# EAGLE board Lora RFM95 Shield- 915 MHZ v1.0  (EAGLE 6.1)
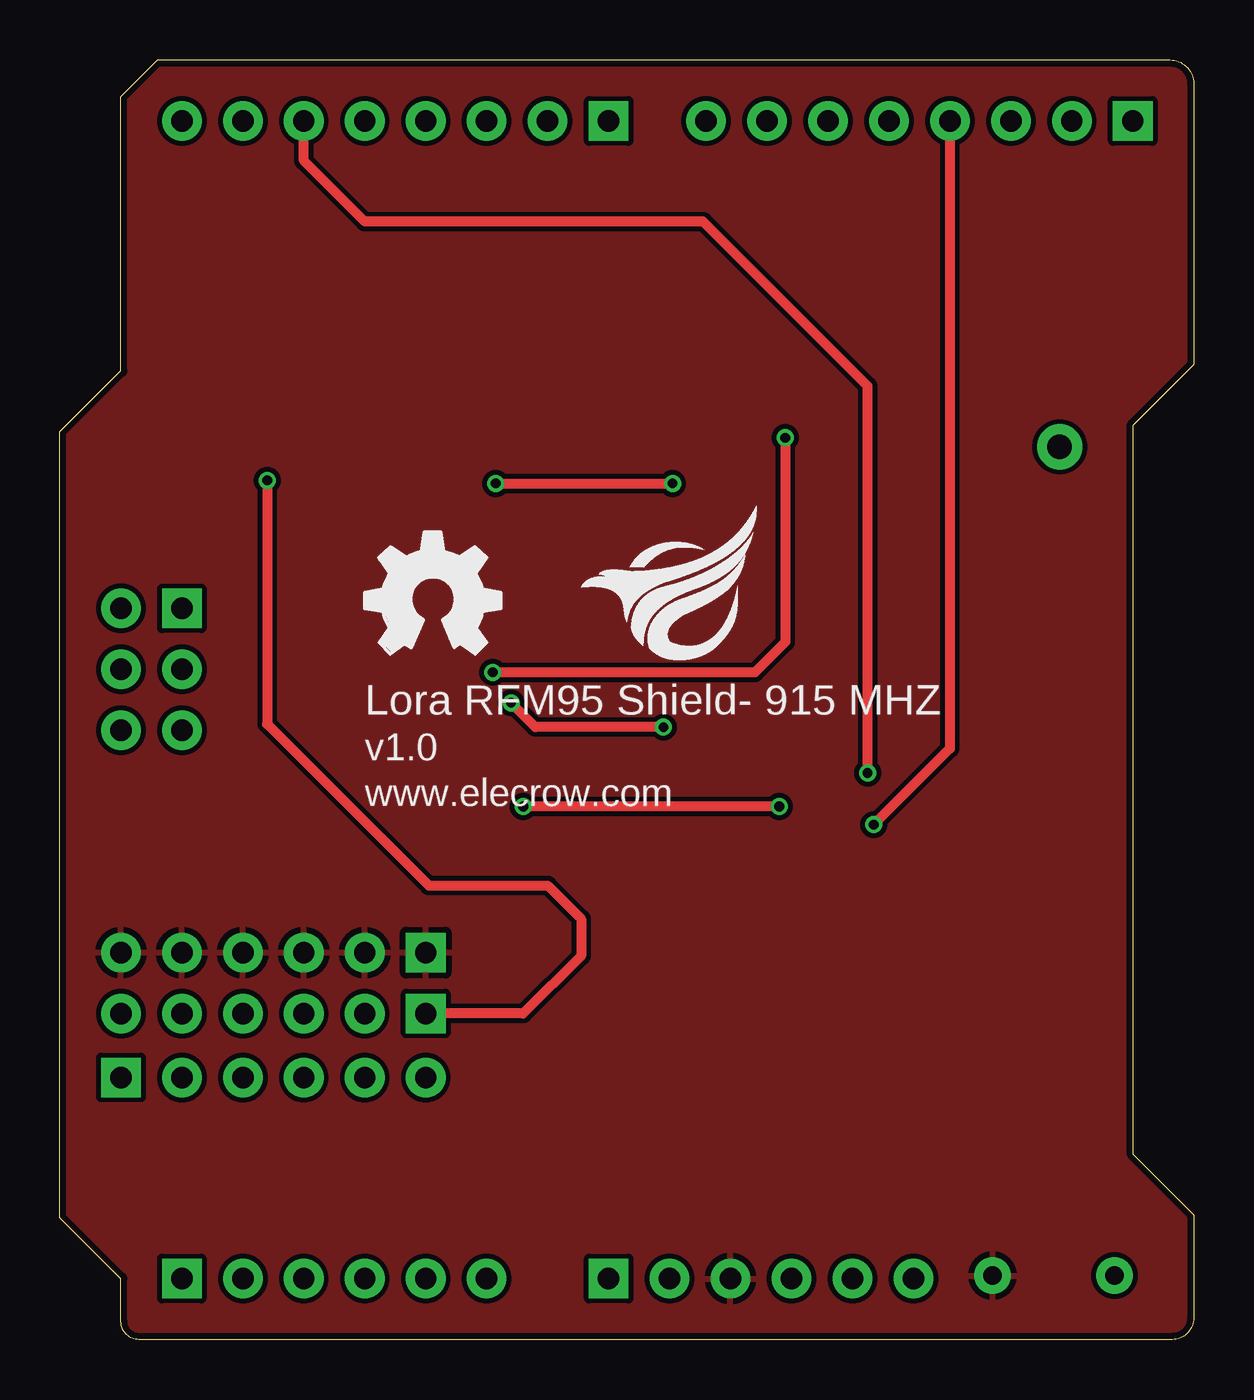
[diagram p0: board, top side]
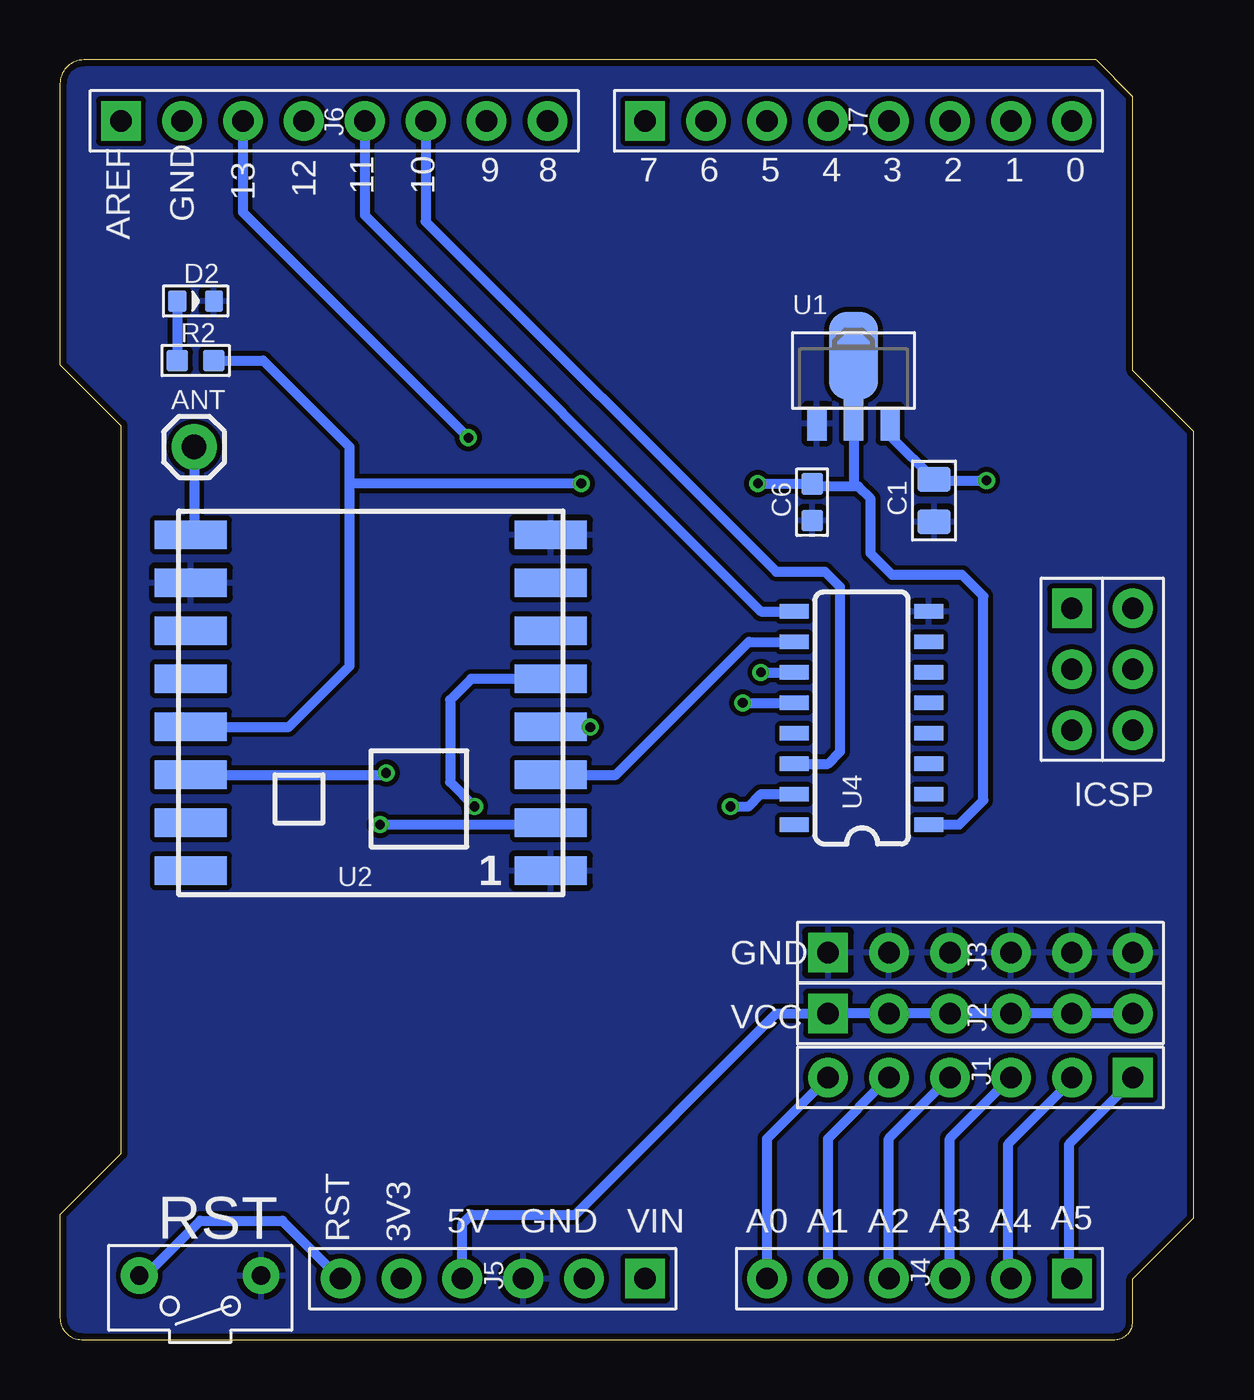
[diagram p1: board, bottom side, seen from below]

Size 47.24 x 53.34 mm. Coordinates in mm from the lower left corner, seen from the top.
Outline: 4.06,53.34 46.25,53.34 arc-90 47.24,52.35 47.24,40.64 44.7,38.1 44.7,7.75 47.24,5.21 47.24,0.9 arc-90 46.35,0 3.28,0 arc-90 2.54,0.74 2.54,2.54 0,5.08 0,37.85 2.54,40.39 2.54,51.82 4.06,53.34
Copper layers (1*16): Top 0.035mm / dielectric 1.5mm / Bottom 0.035mm
Design rules: minimum track width 6mil, minimum drill 12mil, track to track 6mil, track to pad 6mil, pad to pad 6mil, via to via 6mil, smd to smd 0mil, copper to edge 10mil, drill to drill 10mil, minimum pad ring 10mil, minimum via ring 6mil, stop-mask expansion 2mil, vias tented up to drill 100mil, thermal gap 10mil

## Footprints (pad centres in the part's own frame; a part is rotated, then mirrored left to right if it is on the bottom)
1X01 = drill 1.016 pad 1.88: 1 0,0
C0805 = smd 1.016 x 1.397: 1 -0.889,0; 2 0.889,0
C0603 = smd 0.889 x 0.889: 1 -0.762,0; 2 0.762,0
LED-0603 = smd 0.762 x 0.889: + -0.762,0; - 0.762,0
6P-2.54-65/35MIL = drill 0.889 pad 1.651 square: 1 0,6.35 | drill 0.889 pad 1.651: 2 0,3.81; 3 0,1.27; 4 0,-1.27; 5 0,-3.81; 6 0,-6.35
8P-2.54-65/35MIL = drill 0.889 pad 1.651 square: 1 0,8.89 | drill 0.889 pad 1.651: 2 0,6.35; 3 0,3.81; 4 0,1.27; 5 0,-1.27; 6 0,-3.81; 7 0,-6.35; 8 0,-8.89
2X3P-2.54-65/35MIL = drill 0.889 pad 1.651 square: 1 -1.27,2.54 | drill 0.889 pad 1.651: 2 -1.27,0; 3 -1.27,-2.54; 4 1.27,-2.54; 5 1.27,0; 6 1.27,2.54
R0603 = smd 0.889 x 0.889: 1 -0.762,0; 2 0.762,0
2P-7.62X3.56-90D = drill 0.762 pad 1.524: P$1 0,2.54; P$2 0,-2.54
SOT89 = smd 0.8 x 1.4: 1 -1.524,-1.905; 3 1.524,-1.905 | smd 0.8 x 1.9: 2 0,-1.651 | smd 2.032 x 3.65: 4 0,0.94
RFM69HCW-XXXS2 = smd 3 x 1.2: 1 -7.5,7; 2 -7.5,5; 3 -7.5,3; 4 -7.5,1; 5 -7.5,-1; 6 -7.5,-3; 7 -7.5,-5; 8 -7.5,-7; 9 7.5,-7; 10 7.5,-5; 11 7.5,-3; 12 7.5,-1; 13 7.5,1; 14 7.5,3; 15 7.5,5; 16 7.5,7
SO016 = smd 0.6 x 1.2: 1 -4.445,-2.8; 2 -3.175,-2.8; 3 -1.905,-2.8; 4 -0.635,-2.8; 5 0.635,-2.8; 6 1.905,-2.8; 7 3.175,-2.8; 8 4.445,-2.8; 9 4.445,2.8; 10 3.175,2.8; 11 1.905,2.8; 12 0.635,2.8; 13 -0.635,2.8; 14 -1.905,2.8; 15 -3.175,2.8; 16 -4.445,2.8

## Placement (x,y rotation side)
ANT  Antenna  [1X01]  41.66,37.21 0 bottom
C1  10uF  [C0805]  10.82,34.97 90 bottom
C6  0.1uF  [C0603]  15.9,34.91 90 bottom
D2  RED  [LED-0603]  41.59,43.29 0 bottom
J1  [6P-2.54-65/35MIL]  8.89,10.92 270 bottom
J2  [6P-2.54-65/35MIL]  8.89,13.59 90 bottom
J3  [6P-2.54-65/35MIL]  8.89,16.13 90 bottom
J4  [6P-2.54-65/35MIL]  11.43,2.54 270 bottom
J5  [6P-2.54-65/35MIL]  29.21,2.54 270 bottom
J6  [8P-2.54-65/35MIL]  35.81,50.8 90 bottom
J7  [8P-2.54-65/35MIL]  13.97,50.8 90 bottom
J8  [2X3P-2.54-65/35MIL]  3.81,27.94 0 bottom
R2  330  [R0603]  41.59,40.81 0 bottom
RST  K1  [2P-7.62X3.56-90D]  41.4,2.67 270 bottom
U1  [SOT89]  14.18,40.08 0 bottom
U2  RFM69HCW  [RFM69HCW-XXXS2]  34.29,26.54 180 bottom
U4  74HC4050 LVL CONVERTER  [SO016]  13.84,25.91 90 bottom
U$1  [OSHW_FILLX200_NOTEXT]  12.7,28.57 0 top
U$4  [ELECROW_NRW_6]  21.72,28.32 0 top

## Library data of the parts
ANT U4 = SparkFun
C1 C6 D2 R2 RST = Discrete
J1-J8 = Connector
U1 = IC
U2 = mike-temp
U$1 = logo
U$4 = ELECROW

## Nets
3.3V: C6.2 R2.2 U1.2 U1.4 U2.13 U4.1
3V-MOSI: U2.3 U4.10
3V-NSS: U2.5 U4.15
3V-SCK: U2.4 U4.12
5V-MISO: J6.4 U2.2
5V-MOSI: J6.5 U4.9
5V-NSS: J6.6 U4.14
5V-SCK: J6.3 U4.11
DPIO0: J7.6 U2.14
GND: C1.1 C6.1 D2.- J3.1 J3.2 J3.3 J3.4 J3.5 J3.6 J5.3 RST.P$1 U1.1 U2.1 U2.8 U2.10 U4.8
N$1: ANT.1 U2.9
N$2: D2.+ R2.1
N$7: J5.6 RST.P$2
N$10: J5.1
PC0: J1.6 J4.6
PC1: J1.5 J4.5
PC2: J1.4 J4.4
PC3: J1.3 J4.3
PC4: J1.2 J4.2
PC5: J1.1 J4.1
VCC: C1.2 J2.1 J2.2 J2.3 J2.4 J2.5 J2.6 J5.4 U1.3

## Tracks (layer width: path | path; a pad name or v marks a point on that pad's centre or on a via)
3.3V  (via drill 0.41)
  Top 0.406: v18.16,35.69 v25.53,35.69
  Bottom 0.406: U1.4 U1.2 14.18,35.64 14.1,35.56 | 14.1,35.56 13.97,35.56 13.46,35.05 13.46,32.77 12.57,31.88 9.65,31.88 8.76,30.99 8.76,22.48 9.78,21.46 U4.1 | 14.1,35.56 15.79,35.56 C6.2 18.14,35.67 v18.16,35.69 | U2.13 37.7,25.54 35.18,28.07 35.18,35.56 | 35.18,35.56 35.18,37.21 38.78,40.81 R2.2 40.85,40.81 40.89,40.77 | v25.53,35.69 35.05,35.69 35.18,35.56
3V-MOSI
  Bottom 0.406: U2.3 24.08,23.54 18.54,29.08 U4.10
3V-NSS  (via drill 0.41)
  Top 0.406: v29.97,22.23 v19.3,22.23
  Bottom 0.406: U2.5 30.11,27.54 30.99,26.67 30.99,23.24 v29.97,22.23 | v19.3,22.23 18.54,22.23 18.03,22.73 U4.15
3V-SCK  (via drill 0.41)
  Top 0.406: v25.15,25.53 19.81,25.53 v18.8,26.54
  Bottom 0.406: U2.4 25.16,25.54 v25.15,25.53 | v18.8,26.54 U4.12
5V-MISO  (via drill 0.41)
  Top 0.406: J6.4 37.08,24.64 v33.91,21.46
  Bottom 0.406: v33.91,21.46 26.87,21.46 U2.2
5V-MOSI
  Bottom 0.406: J6.5 34.54,46.86 18.03,30.35 U4.9
5V-NSS
  Bottom 0.406: U4.14 15.24,24 14.73,24.51 14.73,31.37 15.37,32 17.4,32 32,46.61 J6.6
5V-SCK  (via drill 0.41)
  Top 0.406: v30.23,37.59 30.23,29.08 28.96,27.81 v18.03,27.81
  Bottom 0.406: 16.51,27.81 U4.11 v18.03,27.81 | J6.3 39.62,46.99 v30.23,37.59
DPIO0  (via drill 0.41)
  Top 0.406: v33.66,23.62 33.66,39.75 26.8,46.61 12.7,46.61 10.16,49.15 J7.6
  Bottom 0.406: U2.14 33.73,23.54 v33.66,23.62
GND
  pour Top (isolate 0.203, rank 6): 47.5,53.34 -0.25,53.34 -0.25,0 47.5,0
  pour Bottom (isolate 0.203, rank 6): 0.51,53.34 -0.13,52.7 -0.13,2.29 2.16,0 47.5,0 47.5,52.7 46.86,53.34
N$1
  Bottom 0.406: ANT.1 41.66,33.4 41.79,33.4 U2.9
N$2
  Bottom 0.406: D2.+ R2.1
N$7
  Bottom 0.406: RST.P$2 43.69,2.67 41.4,4.95 37.97,4.95 J5.6
PC0
  Bottom 0.406: J4.6 17.78,8.38 J1.6
PC1
  Bottom 0.406: J4.5 15.24,8.38 J1.5
PC2
  Bottom 0.406: J4.4 12.7,8.38 J1.4
PC3
  Bottom 0.406: J4.3 10.16,8.38 J1.3
PC4
  Bottom 0.406: J1.2 5.08,10.79 7.75,8.13 7.75,2.67 J4.2
PC5
  Bottom 0.406: J1.1 2.54,10.79 5.21,8.13 5.21,2.67 J4.1
VCC  (via drill 0.41)
  Top 0.406: v8.64,35.81 8.64,25.65 15.37,18.92 20.32,18.92 21.72,17.53 21.72,16 19.3,13.59 J2.1
  Bottom 0.406: U1.3 12.65,37.67 10.82,35.84 | C1.2 10.82,35.84 | 10.82,35.84 10.79,35.81 v8.64,35.81 | J2.6 J2.5 J2.4 J2.3 J2.2 J2.1 17.4,13.59 25.78,5.21 30.1,5.21 30.48,4.83 J5.4

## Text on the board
tPlace: Lora RFM95 Shield- 915 MHZ | v1.0 | www.elecrow.com
bPlace: 0 | 1 | 2 | 3 | 4 | 5 | 6 | 7 | 8 | 9 | 10 | 11 | 12 | 13 | GND | AREF | ICSP | GND | VCC | A5 | A4 | A3 | A2 | A1 | A0 | VIN | GND | 5V | 3V3 | RST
